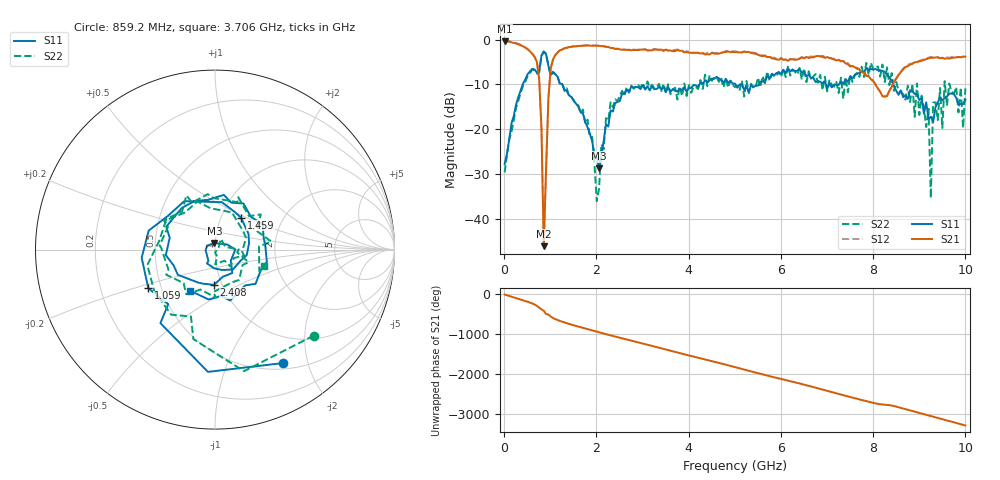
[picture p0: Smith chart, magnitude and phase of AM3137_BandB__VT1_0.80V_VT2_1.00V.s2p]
! Date/Time: Tue, Nov 13, 2018 4:51 PM
! Network Analyzer: Agilent Technologies E8364B Rev: A.07.50.67
! Sweep from 0.010 to 10.000 GHz, 201 Points, Sweep Type: LIN
! Power Supply: 0.800 V, -0.000 A
# Hz S DB R 50
!freq MagS11 AngS11 MagS21 AngS21 MagS12 AngS12 MagS22 AngS22
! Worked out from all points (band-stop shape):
!   201 points, 10 MHz to 10 GHz, reference 50 ohm
!   highest |S21| = -0.36 dB at 10 MHz (marker M1); lowest = -46.1 dB at 859.2 MHz (marker M2)
!   |S21| within 3 dB of the highest: start of sweep to 623.3 MHz; 1.119 GHz to 5.497 GHz (4.378 GHz wide, 132 % of centre)
!   lowest |S11| = -28.7 dB at 2.058 GHz (marker M3), VSWR 1.08, Z = 49.6 + j3.62 ohm
!   |S11| at or under -10 dB: start of sweep to 403.8 MHz; 1.262 GHz to 4.234 GHz (2.971 GHz wide, 108 % of centre); 8.434 GHz to end of sweep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
!   |S22| runs from -36.1 to -2.7 dB; largest |S21 - S12| = 0.026
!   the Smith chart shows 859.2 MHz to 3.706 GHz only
!   S11 on the Smith chart (normalised r, x): 859.2 MHz: 0.58, -1.61; 1.059 GHz: 0.42, -0.22; 1.459 GHz: 1.24, +0.47; 2.408 GHz: 0.92, -0.37; 3.706 GHz: 0.69, -0.34
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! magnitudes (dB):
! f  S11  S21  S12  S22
! 10 MHz  -27.8  -0.4  -0.2  -29.6
! 709.3 MHz  -7.4  -5.0  -4.9  -7.6
! 809.2 MHz  -3.6  -19.8  -19.8  -3.7
! 859.2 MHz  -2.6  -46.1  -45.6  -2.7
! 959 MHz  -5.8  -13.2  -13.2  -5.8
! 1.059 GHz  -7.3  -4.5  -4.4  -7.2
! 1.459 GHz  -12.8  -1.6  -1.6  -12.8
! 1.708 GHz  -16.5  -1.4  -1.3  -15.6
! 2.058 GHz  -28.7  -1.4  -1.3  -33.3
! 2.208 GHz  -18.9  -1.6  -1.6  -17.5
! 2.408 GHz  -14.2  -2.1  -2.0  -13.3
! 3.357 GHz  -10.5  -2.3  -2.2  -9.9
! 3.706 GHz  -11.4  -2.6  -2.4  -10.7
! 5.005 GHz  -9.8  -2.8  -2.6  -10.6
! 6.703 GHz  -8.5  -4.0  -3.8  -8.2
! 8.352 GHz  -8.4  -11.4  -11.4  -10.2
! 9.201 GHz  -17.7  -4.2  -4.0  -15.5
! 9.251 GHz  -17.2  -4.1  -3.9  -35.4
! 9.301 GHz  -18.4  -4.1  -4.0  -14.1
! 9.9 GHz  -14.4  -4.0  -4.0  -10.7
! 9.95 GHz  -14.4  -3.8  -3.8  -19.7
! 10 GHz  -13.4  -3.8  -3.7  -10.9
